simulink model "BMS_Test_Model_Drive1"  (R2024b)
settings: Solver=FixedStepDiscrete  StartTime=0.0  StopTime=inf  FixedStep=0.01  RelTol=1e-3
libraries: nesl_utility x37, fl_lib x35, simulink x31, batteryecm_lib x12, ee_lib x1, SignalEditorBlockLib x1

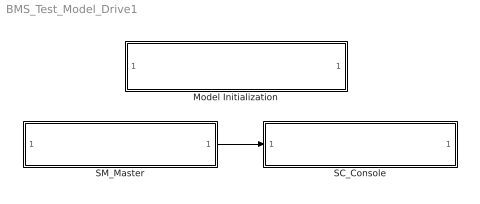
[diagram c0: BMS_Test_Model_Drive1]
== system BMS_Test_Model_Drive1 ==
  Model Initialization : Subsystem  mask(Model Functions){InitFcnX=Ts=0.1;, prel=off, posl=off, inif=off, strf=off}
      mask prompts: InitFcnX "Initialisation"; prel "Preload Function"; posl "PostLoad Function"; inif "InitFcn"; strf "StartFcn"
      mask init:
      | currentBlock = gcb;
      | root = bdroot(currentBlock);
      | 
      | if ~strcmp(get_param(root,'BlockDiagramType'),'library')
      |     if prel==1
      |         set_param(root, 'PreLoadFcn', InitFcnX);
      |     else
      |         set_param(root, 'PreLoadFcn', '');
      |     end
      |     if inif==1
      |         set_param(root, 'InitFcn', InitFcnX);
      |     else
      |         set_param(root, 'InitFcn', '');
      |     end
      |     if strf==1
      |         set_param(root, 'StartFcn', InitFcnX);
      |     else
      |         set_param(root, 'StartFcn', '');
      |     end
      |     if posl==1
      |         set_param(root, 'PostLoadFcn', InitFcnX);
      |     else
      |         set_param(root, 'PostLoadFcn', '');
      |     end
      | end
      | 
      | pos = get_param(currentBlock, 'Position');
      | width = pos(3) - pos(1); height = pos(4) - pos(2);
      | txt = [ upper(root) '\n' '- InitFcn. . . . . '  get_param(root, 'InitFcn') ];
  SC_Console : Subsystem
  SM_Master : Subsystem
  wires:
  SM_Master/1(To_console) -> SC_Console/1(From_Master)

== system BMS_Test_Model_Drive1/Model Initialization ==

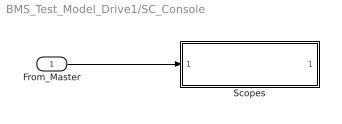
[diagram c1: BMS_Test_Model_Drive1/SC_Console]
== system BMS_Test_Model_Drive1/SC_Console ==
  From_Master : Inport
  Scopes : Subsystem
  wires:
  From_Master/1 -> Scopes/1(From_Master)

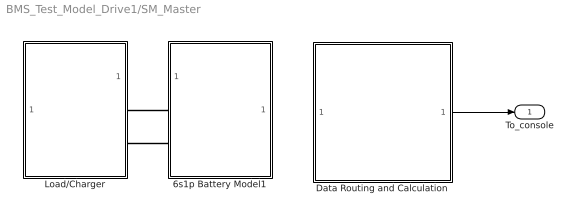
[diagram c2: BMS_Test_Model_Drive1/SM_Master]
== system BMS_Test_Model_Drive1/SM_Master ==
  6s1p Battery Model1 : Subsystem
  Data Routing and Calculation : Subsystem
  Load/Charger : Subsystem
  To_console : Outport
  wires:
  Data Routing and Calculation/1(To Console) -> To_console/1
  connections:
  6s1p Battery Model1/LConn1 -- Load/Charger/RConn1
  6s1p Battery Model1/LConn2 -- Load/Charger/RConn2

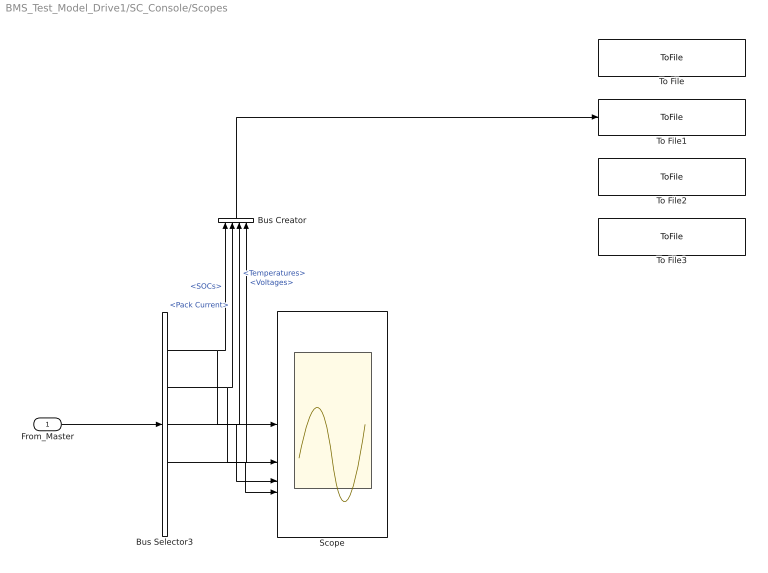
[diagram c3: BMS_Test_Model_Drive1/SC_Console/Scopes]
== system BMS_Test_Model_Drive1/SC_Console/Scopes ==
  From_Master : Inport
  Bus Creator : BusCreator  Inputs=4
  Bus Selector3 : BusSelector  OutputSignals=SOCs,Pack Current,Temperatures,Voltages
  Scope : Scope  NumInputPorts=4
  To File : ToFile  Filename=SimulationUS06_v2.mat  MatrixName=US06_Pack_Data3  SaveFormat=Timeseries
  To File1 : ToFile  Filename=SimulationConstCharge.mat  MatrixName=ConstCharge_Pack_Data3  SaveFormat=Timeseries
  To File2 : ToFile  Filename=SimulationRepeatCharge.mat  MatrixName=RepeatCharge_Pack_Data1  SaveFormat=Timeseries
  To File3 : ToFile  Filename=SimulationBMSSignal.mat  MatrixName=BMSSignal_Pack_Data_Profile2  SaveFormat=Timeseries
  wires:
  From_Master/1 -> Bus Selector3/1
  Bus Selector3/1 -> Bus Creator/1, Scope/1  "<SOCs>"
  Bus Selector3/2 -> Bus Creator/2, Scope/2  "<Pack Current>"
  Bus Selector3/3 -> Bus Creator/3, Scope/3  "<Temperatures>"
  Bus Selector3/4 -> Bus Creator/4, Scope/4  "<Voltages>"
  Bus Creator/1 -> To File1/1

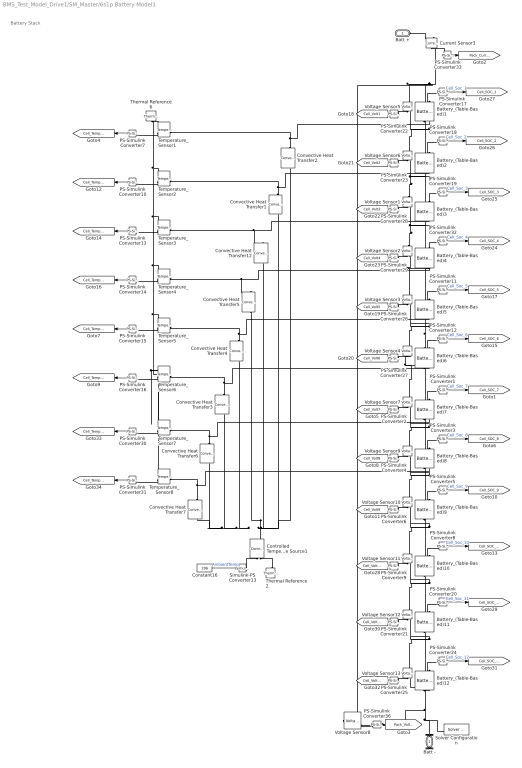
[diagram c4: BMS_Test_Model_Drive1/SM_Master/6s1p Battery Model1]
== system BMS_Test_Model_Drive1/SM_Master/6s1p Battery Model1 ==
  note: Battery Stack
  Battery_(Table-Based){1..12} (12 alike) : batteryecm_lib/Battery (Table-Based)  SOC_vec=[0.04861 0.127807 0.162303 0.2123 0.262472 0.362324 0.462483 0.562334 0.662302 0.762307 0.862372 0.912362 0.962321]  T_dependence=simscape.enum.tablebattery.temperature_dependence.yes  prm_dir=simscape.enum.tablebattery.prm_dir.noCurrentDirectionality  T_vec=[-10 0 25 40 60] degC  V0_mat=[3.225 3.225 3.225 3.225 3.225;3.364 3.364 3.364 3.364 3.364;3.391 3.391 3.391 3.391 3.391;3.451 3.451 3.451 3.451 3.451;3.498 3.498 3.498 3.498 3.498;3.561 3.561 3.561 3.561 3.561;3.622 3.622 3.622 3.622 3.622;3.705 3.705 3.705 3.705 3.705;3.797 3.797 3.797 3.797 3.797;3.882 3.882 3.882 3.882 3.882;3.992 3.992 3.992 3.992 3.992;4.051 4.051 4.051 4.051 4.051;4.102 4.102 4.102 4.102 4.102] V  V0_vec=[3.1, 3.27, 3.31, 3.5] V  V_range=[0, inf] V  R0_mat=[0.169226664942506 0.167163906452554 0.108383589577359 0.166496905009762 0.167551697989061;0.147647439390094 0.12097131496664 0.074350005039498 0.0625868128655119 0.0460556489919985;0.146951059448331 0.118987805825618 0.0728433546029721 0.0628007167120074 0.0489709240971276;0.13307262638046 0.102457131174024 0.0632667622677959 0.0597316704312107 0.0532367466498601;0.123787439191075 0.0935309389464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  R0_vec=[.015, .017, .012, .013] Ohm  R0_dis_mat=[.0117, .0085, .009; .011, .0085, .009; .0114, .0087, .0092; .0107, .0082, .0088; .0107, .0083, .0091; .0113, .0085, .0089; .0116, .0085, .0089] Ohm  R0_dis_vec=[.0085, .0085, .0087, .0082, .0083, .0085, .0085] Ohm  R0_ch_mat=[.0117, .0085, .009; .011, .0085, .009; .0114, .0087, .0092; .0107, .0082, .0088; .0107, .0083, .0091; .0113, .0085, .0089; .0116, .0085, .0089] Ohm  R0_ch_vec=[.0085, .0085, .0087, .0082, .0083, .0085, .0085] Ohm  AH=4.2 hr*A  prm_leak=1  Rleak_vec=[8000, 7000, 6000] Ohm  Rleak=7e3 Ohm  extrapolation_option=simscape.enum.extrapolation.linear  SOC_port=simscape.enum.tablebattery.enable.yes  prm_dyn=1  R1_mat=[0.420596834 0.018909241 0.013850798 0.012242153 0.012242153 0.010862756 0.010747806 0.01138003 0.011724327 0.011839271 0.012126632 0.012242153 0.0137365] Ohm  R1_vec=[.076, .022, .007, .043] Ohm  tau1_mat=[2430 2430 2430 2430 2430 2430 2430 2430 2430 2430 2430 2430 2430] s  tau1_vec=[148, 110, 27, 22] s  R2_mat=[0.353025539 0.018334492 0.006092052 0.007816586 0.005115266 0.005172741 0.006839513 0.004655467 0.004770192 0.007298968 0.007931162 0.005230216 0.005690015] Ohm  R2_vec=[.382, .006, .007, .956] Ohm  tau2_mat=[3550 2410 2420 2430 2420 2420 2430 2420 2430 2420 2430 2422 2421] s  tau2_vec=[44, 24, 14, 13419] s  R3_mat=[.014, .382, .407; .028, .006, .007; .014, .007, .006; .333, .956, .912] Ohm  R3_vec=[.382, .006, .007, .956] Ohm  tau3_mat=[1, 44, 5644; 11, 24, 506; 2, 14, 330; 3310, 13419, 30216] s  tau3_vec=[44, 24, 14, 13419] s  R4_mat=[.014, .382, .407; .028, .006, .007; .014, .007, .006; .333, .956, .912] Ohm  R4_vec=[.382, .006, .007, .956] Ohm  tau4_mat=[1, 44, 5644; 11, 24, 506; 2, 14, 330; 3310, 13419, 30216] s  tau4_vec=[44, 24, 14, 13419] s  R5_mat=[.014, .382, .407; .028, .006, .007; .014, .007, .006; .333, .956, .912] Ohm  R5_vec=[.382, .006, .007, .956] Ohm  tau5_mat=[1, 44, 5644; 11, 24, 506; 2, 14, 330; 3310, 13419, 30216] s  tau5_vec=[44, 24, 14, 13419] s  prm_fade=simscape.enum.tablebattery.prm_fade.disabled  N0=0  dV0=0  dR0=0  dAH=0  dRleak=0  dR1=0  dR2=0  dR3=0  dR4=0  dR5=0  N0vec=[100, 200, 300]  Tfadevec=[298.15, 323.15] K  dV0vec=[0, 0, 0]  dR0vec=[0, 0, 0]  dAHvec=[0, 0, 0]  dRleakvec=[0, 0, 0]  dR1vec=[0, 0, 0]  dR2vec=[0, 0, 0]  dR3vec=[0, 0, 0]  dR4vec=[0, 0, 0]  dR5vec=[0, 0, 0]  dV0mat=[0, 0; 0, 0; 0, 0]  dR0mat=[0, 0; 0, 0; 0, 0]  dAHmat=[0, 0; 0, 0; 0, 0]  dRleakmat=[0, 0; 0, 0; 0, 0]  dR1mat=[0, 0; 0, 0; 0, 0]  dR2mat=[0, 0; 0, 0; 0, 0]  dR3mat=[0, 0; 0, 0; 0, 0]  dR4mat=[0, 0; 0, 0; 0, 0]  dR5mat=[0, 0; 0, 0; 0, 0]  prm_age_modeling=simscape.enum.tablebattery.prm_age_modeling.equation  storage_dt_age_vec=[0] d  storage_T_age_vec=[273] K  prm_age_OCV=simscape.enum.tablebattery.prm_age_OCV.OCV  OCV_age=0.9  SOC_age=0.6  prm_age_resistance=simscape.enum.tablebattery.prm_age.disabled  OCV_scaling_age_resistance=2.2134e6  OCV_offset_age_resistance=1.632e6  temp_exp_age_resistance=0.515833569 V  t_exp_age_resistance=0.75  T_age_vec_resistance=[273.15, 298.15, 323.15] K  dt_age_vec_resistance=[0, 90, 180, 270] d  dR0_age_vec=[0, 0, 0]  t_meas_dR0_age=100 d  dR0_age_mat=[0, 0, 0; 0, 0, 0; 0, 0, 0; 0, 0, 0]  prm_age_capacity=simscape.enum.tablebattery.prm_age.disabled  OCV_scaling_age_capacity=1.5097e07  OCV_offset_age_capacity=8.3625e06  temp_exp_age_capacity=0.6011 V  t_exp_age_capacity=0.75  T_age_vec_capacity=[273.15, 298.15, 323.15] K  dt_age_vec_capacity=[0, 90, 180, 270] d  dAH_age_vec=[0, 0, 0]  t_meas_dAH_age=100 d  dAH_age_mat=[0, 0, 0; 0, 0, 0; 0, 0, 0; 0, 0, 0]  thermal_port=simscape.enum.thermaleffects.model  temperature=296 K  thermal_mass=28 J/K  i_specify=off  i_priority=None  i=0 A  i_nominal_specify=off  i_nominal_value=1  i_nominal_unit=A  v_specify=off  v_priority=High  v=3.657 V  v_nominal_specify=off  v_nominal_value=1  v_nominal_unit=V  stateOfCharge_specify=on  stateOfCharge_priority=High  stateOfCharge=0.05  stateOfCharge_nominal_specify=off  stateOfCharge_nominal_value=1  stateOfCharge_nominal_unit=1  num_cycles_specify=off  num_cycles_priority=High  num_cycles=0  num_cycles_nominal_specify=off  num_cycles_nominal_value=1  num_cycles_nominal_unit=1  cell_temperature_specify=off  cell_temperature_priority=High  cell_temperature=296 K  cell_temperature_nominal_specify=off  cell_temperature_nominal_value=1  cell_temperature_nominal_unit=K
  Constant16 : Constant  Value=296
  Controlled Temperature Source1 : fl_lib/Thermal/Thermal Sources/Controlled Temperature Source
  Convective Heat Transfer{1..7,12} (8 alike) : fl_lib/Thermal/Thermal Elements/Convective Heat Transfer  thermal_type=foundation.enum.constant_variable.constant  area=.00424 m^2  heat_tr_coeff=20 W/(m^2 * K)  min_heat_tr_coeff=1e-3 W/(K*m^2)  T_specify=off  T_priority=None  T=0 K  T_nominal_specify=off  T_nominal_value=1  T_nominal_unit=K  Q_specify=off  Q_priority=None  Q=0 W  Q_nominal_specify=off  Q_nominal_value=1  Q_nominal_unit=W
  Current Sensor3 : fl_lib/Electrical/Electrical Sensors/Current Sensor
  PS-Simulink Converter{1..6,8..9,11..12,17..29,32..33,36} (26 alike) : nesl_utility/PS-Simulink Converter  PhysicalDomain=network_engine_domain  SubClassName=ps_output  LeftPortType=input  RightPortType=output  PseudoPeriodic=off  Frequencies=[]  VectorFormat=1-D array  Unit=1  AffineConversion=off
  PS-Simulink Converter{10,13..16,30..31} (7 alike) : nesl_utility/PS-Simulink Converter  PhysicalDomain=network_engine_domain  SubClassName=ps_output  LeftPortType=input  RightPortType=output  PseudoPeriodic=off  Frequencies=[]  VectorFormat=1-D array  Unit=K  AffineConversion=off
  PS-Simulink Converter7 : nesl_utility/PS-Simulink Converter  PhysicalDomain=network_engine_domain  SubClassName=ps_output  LeftPortType=input  RightPortType=output  PseudoPeriodic=off  Frequencies=[]  VectorFormat=1-D array  Unit=1  AffineConversion=on
  Simulink-PS Converter13 : nesl_utility/Simulink-PS Converter  PhysicalDomain=network_engine_domain  SubClassName=ps_input  LeftPortType=input  RightPortType=output  PseudoPeriodic=off  Frequencies=[]  NoiseDistribution=none  NoiseParameters=[]  Unit=1  AffineConversion=off  FilteringAndDerivatives=provide  SimscapeFilterOrder=1  InputFilterTimeConstant=0.001  UdotUserProvided=0
  Solver Configuration : nesl_utility/Solver Configuration  PhysicalDomain=network_engine_domain  SubClassName=solver  LeftPortType=input  RightPortType=generic  Tones=[]  Harmonics=[]  SimulateNoise=off  Profile=off  UseLocalSampling=off  EnableSwitchedLinearOptims=on  FrequencyDomain=off  UseCCode=off  RelTol=0.001  AbsTol=1e-06  MinStep=1e-09  ToWorkspace=off  RevertToSquareIcSolve=off  NumHomotopyIterations=100  PhasorMode=off  PhasorModeNumHarmonics=1  ConsistencySolver=NEWTON_FTOL  IndexReductionMethod=DerivativeReplacement  DoDC=off  ResidualTolerance=1e-09  ConsistencyTolSource=GLOBAL  ConsistencyAbsTol=0.001  ConsistencyRelTol=0.001  ConsistencyTolFactor=0.001  UseLocalSolver=on  LocalSolverChoice=NE_BACKWARD_EULER_ADVANCER  ResolveIndetEquations=on  FunctionEvalNumThread=1  LocalSolverSampleTime=0.25  DoFixedCost=on  MaxNonlinIter=3  MaxModeIter=2  ComputeImpulses=off  ImpulseIterations=2  LinearAlgebra=auto  LinearAlgebraNumThread=0  EquationFormulation=NE_TIME_EF  DelaysMemoryBudget=1024  AutomaticFiltering=on  FilteringTimeConstant=0.001  PartitionStorageMethod=AS_NEEDED  PartitionMemoryBudget=1024  PartitionMethod=FAST  MultibodyUseLocalSolver=off  MultibodyLocalSolverChoice=ODE1  MultibodyLocalSolverSampleTime=0.001
  Temperature_Sensor{1..8} (8 alike) : fl_lib/Thermal/Thermal Sensors/Temperature Sensor  temperature_measure=foundation.enum.MeasurementReference.difference
  Thermal Reference2 : fl_lib/Thermal/Thermal Elements/Thermal Reference
  Thermal Reference6 : fl_lib/Thermal/Thermal Elements/Thermal Reference
  Voltage Sensor{1..13} (13 alike) : fl_lib/Electrical/Electrical Sensors/Voltage Sensor
  Batt + : PMIOPort  Side=Left
  Batt - : PMIOPort  Port=2  Side=Left
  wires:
  PS-Simulink Converter33/1 -> [Pack_Current]
  PS-Simulink Converter36/1 -> [Pack_Voltage]
  PS-Simulink Converter27/1 -> [Cell_Volt6]
  PS-Simulink Converter23/1 -> [Cell_Volt2]
  PS-Simulink Converter28/1 -> [Cell_Volt3]
  PS-Simulink Converter26/1 -> [Cell_Volt5]
  PS-Simulink Converter22/1 -> [Cell_Volt1]
  PS-Simulink Converter29/1 -> [Cell_Volt4]
  PS-Simulink Converter7/1 -> [Cell_Temp_1_k]
  PS-Simulink Converter10/1 -> [Cell_Temp_2_k]
  PS-Simulink Converter13/1 -> [Cell_Temp_3_k]
  PS-Simulink Converter14/1 -> [Cell_Temp_4_k]
  PS-Simulink Converter15/1 -> [Cell_Temp_5_k]
  PS-Simulink Converter16/1 -> [Cell_Temp_6_k]
  PS-Simulink Converter12/1 -> [Cell_SOC_6]  "Cell_Soc_6"
  PS-Simulink Converter11/1 -> [Cell_SOC_5]  "Cell_Soc_5"
  PS-Simulink Converter32/1 -> [Cell_SOC_4]  "Cell_Soc_4"
  PS-Simulink Converter19/1 -> [Cell_SOC_3]  "Cell_Soc_3"
  PS-Simulink Converter18/1 -> [Cell_SOC_2]  "Cell_Soc_2"
  PS-Simulink Converter17/1 -> [Cell_SOC_1]  "Cell_Soc_1"
  PS-Simulink Converter1/1 -> [Cell_SOC_7]  "Cell_Soc_7"
  PS-Simulink Converter2/1 -> [Cell_Volt7]
  PS-Simulink Converter4/1 -> [Cell_Volt8]
  PS-Simulink Converter3/1 -> [Cell_SOC_8]  "Cell_Soc_8"
  PS-Simulink Converter5/1 -> [Cell_SOC_9]  "Cell_Soc_9"
  PS-Simulink Converter6/1 -> [Cell_Volt9]
  PS-Simulink Converter8/1 -> [Cell_SOC_10]  "Cell_Soc_10"
  PS-Simulink Converter9/1 -> [Cell_Volt10]
  PS-Simulink Converter21/1 -> [Cell_Volt11]
  PS-Simulink Converter20/1 -> [Cell_SOC_11]  "Cell_Soc_11"
  PS-Simulink Converter24/1 -> [Cell_SOC_12]  "Cell_Soc_12"
  PS-Simulink Converter25/1 -> [Cell_Volt12]
  PS-Simulink Converter30/1 -> [Cell_Temp_7_k]
  PS-Simulink Converter31/1 -> [Cell_Temp_8_k]
  Constant16/1 -> Simulink-PS Converter13/1  "AmbientTemp"
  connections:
  Temperature_Sensor3/LConn1 -- Battery_(Table-Based)3/RConn2 -- Convective Heat Transfer12/RConn1
  Convective Heat Transfer5/LConn1 -- Convective Heat Transfer7/LConn1 -- Convective Heat Transfer6/LConn1 -- Convective Heat Transfer3/LConn1 -- Convective Heat Transfer4/LConn1 -- Convective Heat Transfer2/LConn1 -- Convective Heat Transfer1/LConn1 -- Convective Heat Transfer12/LConn1 -- Controlled Temperature Source1/LConn1
  Battery_(Table-Based)6/LConn1 -- Voltage Sensor4/LConn1 -- Voltage Sensor3/RConn2 -- Battery_(Table-Based)5/RConn1
  Temperature_Sensor4/LConn1 -- Battery_(Table-Based)4/RConn2 -- Convective Heat Transfer5/RConn1
  Voltage Sensor2/RConn2 -- Voltage Sensor3/LConn1 -- Battery_(Table-Based)4/RConn1 -- Battery_(Table-Based)5/LConn1
  Convective Heat Transfer3/RConn1 -- Battery_(Table-Based)6/RConn2 -- Temperature_Sensor6/LConn1
  Battery_(Table-Based)1/RConn1 -- Voltage Sensor6/LConn1 -- Voltage Sensor5/RConn2 -- Battery_(Table-Based)2/LConn1
  Convective Heat Transfer4/RConn1 -- Battery_(Table-Based)5/RConn2 -- Temperature_Sensor5/LConn1
  Convective Heat Transfer1/RConn1 -- Battery_(Table-Based)2/RConn2 -- Temperature_Sensor2/LConn1
  Convective Heat Transfer2/RConn1 -- Battery_(Table-Based)1/RConn2 -- Temperature_Sensor1/LConn1
  PS-Simulink Converter11/LConn1 -- Battery_(Table-Based)5/LConn2
  Temperature_Sensor5/RConn2 -- PS-Simulink Converter15/LConn1
  Temperature_Sensor6/RConn2 -- PS-Simulink Converter16/LConn1
  PS-Simulink Converter12/LConn1 -- Battery_(Table-Based)6/LConn2
  PS-Simulink Converter18/LConn1 -- Battery_(Table-Based)2/LConn2
  PS-Simulink Converter17/LConn1 -- Battery_(Table-Based)1/LConn2
  Temperature_Sensor3/RConn2 -- PS-Simulink Converter13/LConn1
  Simulink-PS Converter13/RConn1 -- Controlled Temperature Source1/RConn1
  Thermal Reference6/LConn1 -- Temperature_Sensor1/RConn1 -- Temperature_Sensor2/RConn1 -- Temperature_Sensor3/RConn1 -- Temperature_Sensor4/RConn1 -- Temperature_Sensor5/RConn1 -- Temperature_Sensor8/RConn1 -- Temperature_Sensor7/RConn1 -- Temperature_Sensor6/RConn1
  Battery_(Table-Based)4/LConn2 -- PS-Simulink Converter32/LConn1
  Thermal Reference2/LConn1 -- Controlled Temperature Source1/RConn2
  Battery_(Table-Based)3/LConn2 -- PS-Simulink Converter19/LConn1
  Temperature_Sensor4/RConn2 -- PS-Simulink Converter14/LConn1
  Temperature_Sensor2/RConn2 -- PS-Simulink Converter10/LConn1
  Temperature_Sensor1/RConn2 -- PS-Simulink Converter7/LConn1
  Voltage Sensor8/LConn1 -- Voltage Sensor5/LConn1 -- Battery_(Table-Based)1/LConn1 -- Current Sensor3/RConn2
  Battery_(Table-Based)6/RConn1 -- Battery_(Table-Based)7/LConn1 -- Voltage Sensor7/LConn1 -- Voltage Sensor4/RConn2
  Batt +/RConn1 -- Current Sensor3/LConn1
  PS-Simulink Converter33/LConn1 -- Current Sensor3/RConn1
  PS-Simulink Converter27/LConn1 -- Voltage Sensor4/RConn1
  PS-Simulink Converter28/LConn1 -- Voltage Sensor1/RConn1
  PS-Simulink Converter29/LConn1 -- Voltage Sensor2/RConn1
  PS-Simulink Converter23/LConn1 -- Voltage Sensor6/RConn1
  PS-Simulink Converter26/LConn1 -- Voltage Sensor3/RConn1
  PS-Simulink Converter22/LConn1 -- Voltage Sensor5/RConn1
  Voltage Sensor2/LConn1 -- Battery_(Table-Based)4/LConn1 -- Battery_(Table-Based)3/RConn1 -- Voltage Sensor1/RConn2
  Voltage Sensor1/LConn1 -- Battery_(Table-Based)3/LConn1 -- Battery_(Table-Based)2/RConn1 -- Voltage Sensor6/RConn2
  Voltage Sensor8/RConn1 -- PS-Simulink Converter36/LConn1
  Battery_(Table-Based)7/RConn1 -- Voltage Sensor9/LConn1 -- Voltage Sensor7/RConn2 -- Battery_(Table-Based)8/LConn1
  PS-Simulink Converter2/LConn1 -- Voltage Sensor7/RConn1
  PS-Simulink Converter1/LConn1 -- Battery_(Table-Based)7/LConn2
  Battery_(Table-Based)12/RConn1 -- Voltage Sensor13/RConn2 -- Voltage Sensor8/RConn2 -- Solver Configuration/RConn1 -- Batt -/RConn1
  Battery_(Table-Based)8/RConn1 -- Voltage Sensor10/LConn1 -- Voltage Sensor9/RConn2 -- Battery_(Table-Based)9/LConn1
  PS-Simulink Converter3/LConn1 -- Battery_(Table-Based)8/LConn2
  PS-Simulink Converter4/LConn1 -- Voltage Sensor9/RConn1
  Battery_(Table-Based)9/RConn1 -- Voltage Sensor11/LConn1 -- Voltage Sensor10/RConn2 -- Battery_(Table-Based)10/LConn1
  PS-Simulink Converter5/LConn1 -- Battery_(Table-Based)9/LConn2
  PS-Simulink Converter6/LConn1 -- Voltage Sensor10/RConn1
  Battery_(Table-Based)10/RConn1 -- Voltage Sensor12/LConn1 -- Voltage Sensor11/RConn2 -- Battery_(Table-Based)11/LConn1
  PS-Simulink Converter8/LConn1 -- Battery_(Table-Based)10/LConn2
  PS-Simulink Converter9/LConn1 -- Voltage Sensor11/RConn1
  Battery_(Table-Based)11/RConn1 -- Voltage Sensor13/LConn1 -- Voltage Sensor12/RConn2 -- Battery_(Table-Based)12/LConn1
  PS-Simulink Converter20/LConn1 -- Battery_(Table-Based)11/LConn2
  PS-Simulink Converter21/LConn1 -- Voltage Sensor12/RConn1
  PS-Simulink Converter25/LConn1 -- Voltage Sensor13/RConn1
  PS-Simulink Converter24/LConn1 -- Battery_(Table-Based)12/LConn2
  Temperature_Sensor7/RConn2 -- PS-Simulink Converter30/LConn1
  Convective Heat Transfer6/RConn1 -- Battery_(Table-Based)7/RConn2 -- Temperature_Sensor7/LConn1
  Convective Heat Transfer7/RConn1 -- Battery_(Table-Based)8/RConn2 -- Temperature_Sensor8/LConn1
  Temperature_Sensor8/RConn2 -- PS-Simulink Converter31/LConn1

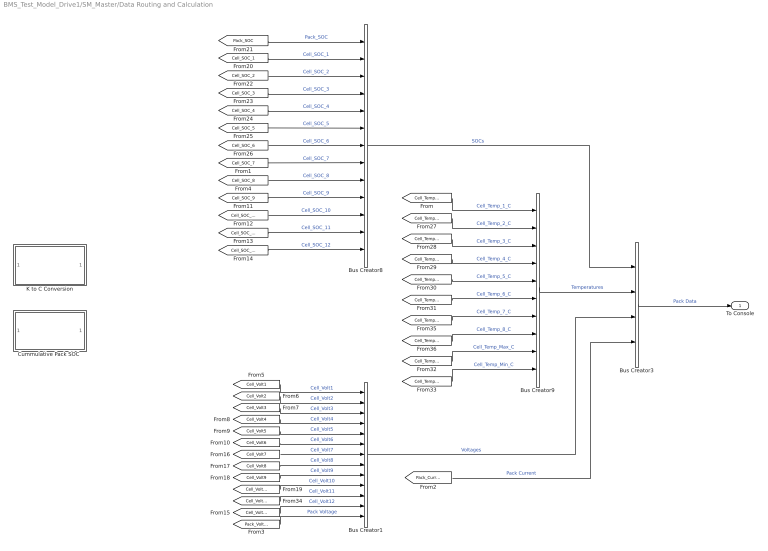
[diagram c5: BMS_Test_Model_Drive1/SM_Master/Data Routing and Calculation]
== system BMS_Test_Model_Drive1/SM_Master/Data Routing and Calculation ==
  Bus Creator1 : BusCreator  Inputs=13
  Bus Creator3 : BusCreator  Inputs=4
  Bus Creator8 : BusCreator  Inputs=13
  Bus Creator9 : BusCreator  Inputs=10
  "Cummulative Pack SOC " : Subsystem
  K to C Conversion : Subsystem
  To Console : Outport  VectorParamsAs1DForOutWhenUnconnected=off
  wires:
  [Cell_Volt3] -> Bus Creator1/3  "Cell_Volt3"
  [Cell_Volt1] -> Bus Creator1/1  "Cell_Volt1"
  [Cell_Volt2] -> Bus Creator1/2  "Cell_Volt2"
  [Cell_Volt5] -> Bus Creator1/5  "Cell_Volt5"
  [Cell_Volt6] -> Bus Creator1/6  "Cell_Volt6"
  [Cell_Volt4] -> Bus Creator1/4  "Cell_Volt4"
  Bus Creator3/1 -> To Console/1  "Pack Data"
  [Pack_SOC] -> Bus Creator8/1  "Pack_SOC"
  [Cell_SOC_1] -> Bus Creator8/2  "Cell_SOC_1"
  [Cell_SOC_2] -> Bus Creator8/3  "Cell_SOC_2"
  [Cell_SOC_3] -> Bus Creator8/4  "Cell_SOC_3"
  [Cell_SOC_4] -> Bus Creator8/5  "Cell_SOC_4"
  [Cell_SOC_5] -> Bus Creator8/6  "Cell_SOC_5"
  [Cell_SOC_6] -> Bus Creator8/7  "Cell_SOC_6"
  Bus Creator8/1 -> Bus Creator3/1  "SOCs"
  [Cell_Temp_1_C] -> Bus Creator9/1  "Cell_Temp_1_C"
  [Cell_Temp_2_C] -> Bus Creator9/2  "Cell_Temp_2_C"
  [Cell_Temp_3_C] -> Bus Creator9/3  "Cell_Temp_3_C"
  [Cell_Temp_4_C] -> Bus Creator9/4  "Cell_Temp_4_C"
  [Cell_Temp_5_C] -> Bus Creator9/5  "Cell_Temp_5_C"
  [Cell_Temp_6_C] -> Bus Creator9/6  "Cell_Temp_6_C"
  [Cell_Temp_Max_C] -> Bus Creator9/9  "Cell_Temp_Max_C"
  [Cell_Temp_Min_C] -> Bus Creator9/10  "Cell_Temp_Min_C"
  [Pack_Current] -> Bus Creator3/4  "Pack Current"
  Bus Creator9/1 -> Bus Creator3/2  "Temperatures"
  Bus Creator1/1 -> Bus Creator3/3  "Voltages"
  [Cell_SOC_7] -> Bus Creator8/8  "Cell_SOC_7"
  [Cell_SOC_8] -> Bus Creator8/9  "Cell_SOC_8"
  [Cell_SOC_9] -> Bus Creator8/10  "Cell_SOC_9"
  [Cell_SOC_10] -> Bus Creator8/11  "Cell_SOC_10"
  [Cell_SOC_11] -> Bus Creator8/12  "Cell_SOC_11"
  [Cell_SOC_12] -> Bus Creator8/13  "Cell_SOC_12"
  [Pack_Voltage] -> Bus Creator1/13  "Pack Voltage"
  [Cell_Volt7] -> Bus Creator1/7  "Cell_Volt7"
  [Cell_Volt8] -> Bus Creator1/8  "Cell_Volt8"
  [Cell_Volt9] -> Bus Creator1/9  "Cell_Volt9"
  [Cell_Volt10] -> Bus Creator1/10  "Cell_Volt10"
  [Cell_Volt11] -> Bus Creator1/11  "Cell_Volt11"
  [Cell_Volt12] -> Bus Creator1/12  "Cell_Volt12"
  [Cell_Temp_7_C] -> Bus Creator9/7  "Cell_Temp_7_C"
  [Cell_Temp_8_C] -> Bus Creator9/8  "Cell_Temp_8_C"

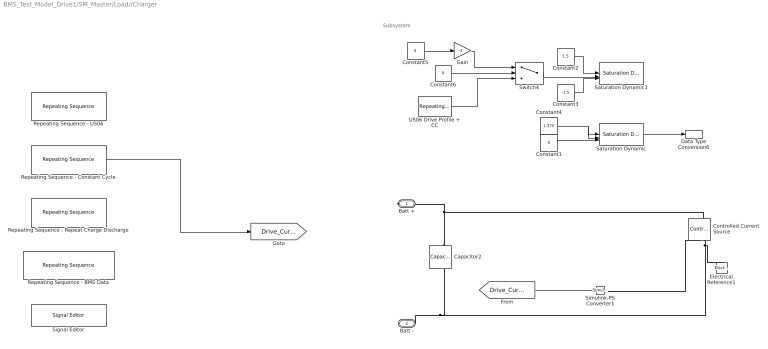
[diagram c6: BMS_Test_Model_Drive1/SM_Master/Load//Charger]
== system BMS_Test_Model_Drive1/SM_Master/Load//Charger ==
  note: Subsystem
  Capacitor2 : ee_lib/Passive/Capacitor  cap_option=ee.enum.passive.capacitor.capOption.const  c=1e-6 F  Cvec=[1e-05, 1e-06] F  Vvec=[0, 10] V  CV_table_symmetry=1  f_vec=[1, 10] kHz  DFext_vec=[.8, 1.2]  enable_C_tol=0  averaging_period=0 s  C_tol=5  tol_distribution=1  nSigma=4  r=1e-6 Ohm  g=0 1/Ohm  enable_operating_limits=0  operating_limit_action=2  max_working_voltage_range=[-25, 25] V  power_rating=1 W  maxTemperature=85 degC  thermalEnable=false  thermalMass=1 J/K  fault_action=simscape.enum.assert.action.none  t_fault=1 s  i_specify=off  i_priority=None  i=0 A  i_nominal_specify=off  i_nominal_value=1  i_nominal_unit=A  v_specify=off  v_priority=None  v=0 V  v_nominal_specify=off  v_nominal_value=1  v_nominal_unit=V  vc_specify=on  vc_priority=High  vc=0 V  vc_nominal_specify=off  vc_nominal_value=1  vc_nominal_unit=V  T_specify=off  T_priority=None  T=298.15 K  T_nominal_specify=off  T_nominal_value=1  T_nominal_unit=K
  Constant1 : Constant  Commented=on  Value=0
  Constant2 : Constant  Commented=on  Value=1.5
  Constant3 : Constant  Commented=on  Value=-1.5
  Constant4 : Constant  Commented=on  Value=1.375
  Constant5 : Constant  Commented=on  Value=0
  Constant6 : Constant  Commented=on  Value=0
  Controlled Current Source : fl_lib/Electrical/Electrical Sources/Controlled Current Source
  Data Type Conversion6 : DataTypeConversion  Commented=on
  Electrical Reference1 : fl_lib/Electrical/Electrical Elements/Electrical Reference
  Gain : Gain  Commented=on  Gain=-1
  Repeating Sequence - BMS Data : simulink/Sources/Repeating Sequence  Commented=on  rep_seq_t=time_monotonic  rep_seq_y=current_vector
  Repeating Sequence - Constant Cycle : simulink/Sources/Repeating Sequence  rep_seq_t=time_monotonic  rep_seq_y=current_vector
  Repeating Sequence - Repeat Charge Discharge : simulink/Sources/Repeating Sequence  Commented=on  rep_seq_t=time_monotonic  rep_seq_y=current_vector
  Repeating Sequence - US06 : simulink/Sources/Repeating Sequence  Commented=on  rep_seq_t=time_monotonic  rep_seq_y=current_US06
  Saturation Dynamic : simulink/Discontinuities/Saturation Dynamic  Commented=on  OutMin=[]  OutMax=[]  OutDataTypeStr=Inherit: Same as second input  OutDataType=fixdt(1, 16)  OutScaling=2^-10  DoSatur=off
  Saturation Dynamic1 : simulink/Discontinuities/Saturation Dynamic  Commented=on  OutMin=[]  OutMax=[]  OutDataTypeStr=Inherit: Same as second input  OutDataType=fixdt(1, 16)  OutScaling=2^-10  DoSatur=off
  Signal Editor : SignalEditorBlockLib/Signal Editor  Commented=on  FileName=currentSignal.mat  ActiveScenario=Scenario  ActiveSignal=currentSignal  IsBus=off  OutputBusObjectStr=Bus: BusObject  SampleTime=0  Interpolate=off  ZeroCross=off  OutputAfterFinalValue=Setting to zero  Unit=inherit  PreserveSignalName=on  ApplySigPropsToAllScenarios=on  ApplySigPropsToAllSignals=off
  Simulink-PS Converter1 : nesl_utility/Simulink-PS Converter  PhysicalDomain=network_engine_domain  SubClassName=ps_input  LeftPortType=input  RightPortType=output  PseudoPeriodic=off  Frequencies=[]  NoiseDistribution=none  NoiseParameters=[]  Unit=1  AffineConversion=off  FilteringAndDerivatives=provide  SimscapeFilterOrder=1  InputFilterTimeConstant=0.001  UdotUserProvided=0
  Switch4 : Switch  Commented=on  Criteria=u2 > Threshold
  US06 Drive Profile + CC : simulink/Sources/Repeating Sequence  Commented=on  rep_seq_t=[0 1 2]  rep_seq_y=[0 0 0]
  Batt + : PMIOPort  Side=Right
  Batt - : PMIOPort  Port=2  Side=Right
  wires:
  US06 Drive Profile + CC/1 -> Switch4/3
  Gain/1 -> Switch4/1
  Constant3/1 -> Saturation Dynamic1/3
  Constant5/1 -> Gain/1
  Constant2/1 -> Saturation Dynamic1/1
  Constant6/1 -> Switch4/2
  Switch4/1 -> Saturation Dynamic1/2
  Data Type Conversion6/1 -> ?
  Constant1/1 -> Saturation Dynamic/3
  Constant4/1 -> Saturation Dynamic/2, Saturation Dynamic/1
  Saturation Dynamic/1 -> Data Type Conversion6/1
  Saturation Dynamic1/1 -> ?
  [Drive_Current] -> Simulink-PS Converter1/1
  Repeating Sequence - Constant Cycle/1 -> [Drive_Current]
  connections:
  Capacitor2/LConn1 -- Batt +/RConn1 -- Controlled Current Source/LConn1
  Simulink-PS Converter1/RConn1 -- Controlled Current Source/RConn1
  Controlled Current Source/RConn2 -- Electrical Reference1/LConn1 -- Capacitor2/RConn1 -- Batt -/RConn1

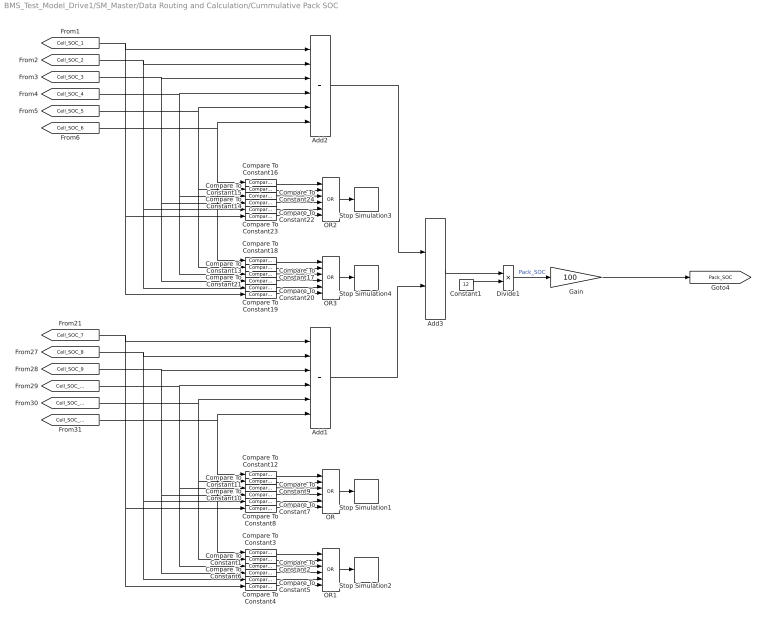
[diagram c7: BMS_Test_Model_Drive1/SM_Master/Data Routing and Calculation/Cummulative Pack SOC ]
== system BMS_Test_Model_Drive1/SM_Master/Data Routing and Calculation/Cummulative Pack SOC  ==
  Add1 : Sum  Inputs=++++++
  Add2 : Sum  Inputs=++++++
  Add3 : Sum
  Compare To Constant{1..6,13,17..21} (12 alike) : simulink/Logic and Bit Operations/Compare To Constant  relop=>=  const=1  OutDataTypeStr=boolean
  Compare To Constant{7..12,14..16,22..24} (12 alike) : simulink/Logic and Bit Operations/Compare To Constant  relop=<=  const=0.001  OutDataTypeStr=boolean
  Constant1 : Constant  Value=12
  Divide1 : Product  Inputs=*/
  Gain : Gain  Gain=100
  OR{,1..3} (4 alike) : Logic  Operator=OR  Inputs=6  IconShape=distinctive  AllPortsSameDT=off  OutDataTypeStr=boolean
  Stop Simulation{1..4} (4 alike) : Stop
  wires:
  [Cell_SOC_10] -> Compare To Constant2/1, Compare To Constant9/1, Add1/4
  [Cell_SOC_7] -> Compare To Constant5/1, Compare To Constant7/1, Add1/1
  [Cell_SOC_9] -> Compare To Constant6/1, Compare To Constant10/1, Add1/3
  [Cell_SOC_8] -> Compare To Constant4/1, Compare To Constant8/1, Add1/2
  [Cell_SOC_12] -> Compare To Constant3/1, Compare To Constant12/1, Add1/6
  [Cell_SOC_11] -> Compare To Constant1/1, Compare To Constant11/1, Add1/5
  Compare To Constant5/1 -> OR1/6
  Compare To Constant8/1 -> OR/5
  Compare To Constant11/1 -> OR/2
  Compare To Constant9/1 -> OR/3
  Compare To Constant3/1 -> OR1/1
  Compare To Constant2/1 -> OR1/3
  Compare To Constant10/1 -> OR/4
  OR1/1 -> Stop Simulation2/1
  Compare To Constant6/1 -> OR1/4
  Compare To Constant7/1 -> OR/6
  Compare To Constant1/1 -> OR1/2
  Compare To Constant12/1 -> OR/1
  Compare To Constant4/1 -> OR1/5
  OR/1 -> Stop Simulation1/1
  [Cell_SOC_5] -> Compare To Constant13/1, Compare To Constant15/1, Add2/5
  Compare To Constant15/1 -> OR2/2
  Compare To Constant13/1 -> OR3/2
  OR3/1 -> Stop Simulation4/1
  [Cell_SOC_6] -> Compare To Constant18/1, Compare To Constant16/1, Add2/6
  [Cell_SOC_4] -> Compare To Constant17/1, Compare To Constant24/1, Add2/4
  Compare To Constant18/1 -> OR3/1
  Compare To Constant24/1 -> OR2/3
  Constant1/1 -> Divide1/2
  Compare To Constant16/1 -> OR2/1
  [Cell_SOC_1] -> Compare To Constant20/1, Compare To Constant22/1, Add2/1
  [Cell_SOC_3] -> Compare To Constant21/1, Compare To Constant14/1, Add2/3
  Compare To Constant19/1 -> OR3/5
  [Cell_SOC_2] -> Compare To Constant19/1, Compare To Constant23/1, Add2/2
  Compare To Constant21/1 -> OR3/4
  Compare To Constant14/1 -> OR2/4
  Compare To Constant22/1 -> OR2/6
  Compare To Constant20/1 -> OR3/6
  OR2/1 -> Stop Simulation3/1
  Compare To Constant23/1 -> OR2/5
  Compare To Constant17/1 -> OR3/3
  Add3/1 -> Divide1/1
  Add2/1 -> Add3/1
  Add1/1 -> Add3/2
  Divide1/1 -> Gain/1  "Pack_SOC"
  Gain/1 -> [Pack_SOC]

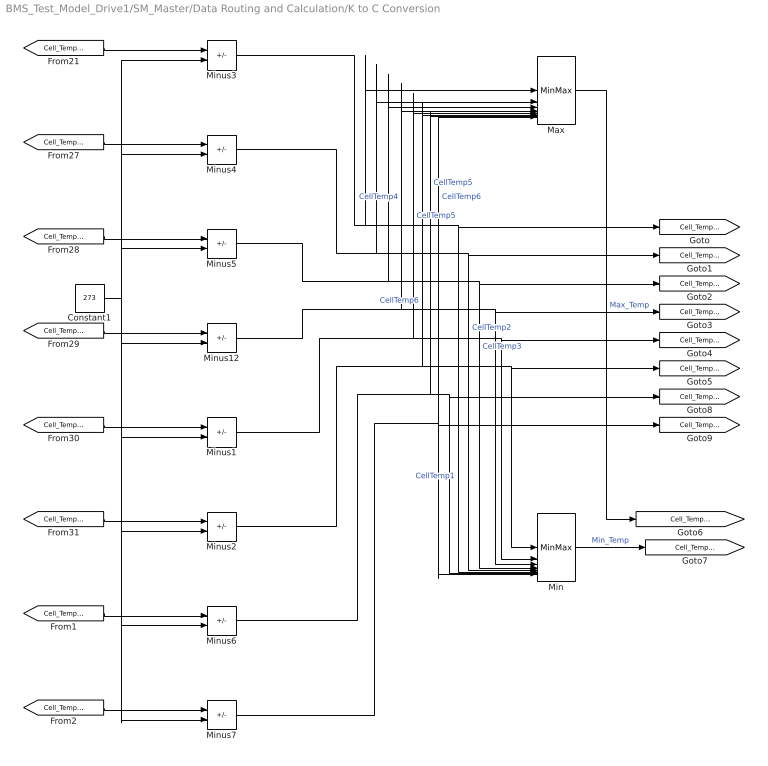
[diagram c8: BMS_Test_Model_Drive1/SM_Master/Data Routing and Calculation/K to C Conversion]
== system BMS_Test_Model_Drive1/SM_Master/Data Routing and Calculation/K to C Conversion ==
  Constant1 : Constant  Value=273
  Max : MinMax  Function=max  Inputs=8
  Min : MinMax  Inputs=8
  Minus{1..7,12} (8 alike) : Sum  Inputs=+-
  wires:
  [Cell_Temp_1_k] -> Minus3/1
  Max/1 -> [Cell_Temp_Max_C]  "Max_Temp"
  Minus3/1 -> [Cell_Temp_1_C], Min/6, Max/1  "CellTemp1"
  [Cell_Temp_2_k] -> Minus4/1
  [Cell_Temp_6_k] -> Minus2/1
  Min/1 -> [Cell_Temp_Min_C]  "Min_Temp"
  Minus12/1 -> [Cell_Temp_4_C], Min/3, Max/4  "CellTemp4"
  Constant1/1 -> Minus7/2, Minus6/2, Minus2/2, Minus1/2, Minus12/2, Minus5/2, Minus4/2, Minus3/2
  [Cell_Temp_4_k] -> Minus12/1
  Minus2/1 -> [Cell_Temp_6_C], Min/1, Max/6  "CellTemp6"
  [Cell_Temp_5_k] -> Minus1/1
  Minus1/1 -> [Cell_Temp_5_C], Min/2, Max/5  "CellTemp5"
  Minus4/1 -> [Cell_Temp_2_C], Min/5, Max/2  "CellTemp2"
  [Cell_Temp_3_k] -> Minus5/1
  Minus5/1 -> [Cell_Temp_3_C], Min/4, Max/3  "CellTemp3"
  [Cell_Temp_7_k] -> Minus6/1
  [Cell_Temp_8_k] -> Minus7/1
  Minus6/1 -> Max/7, Min/7, [Cell_Temp_7_C]  "CellTemp5"
  Minus7/1 -> Min/8, Max/8, [Cell_Temp_8_C]  "CellTemp6"
